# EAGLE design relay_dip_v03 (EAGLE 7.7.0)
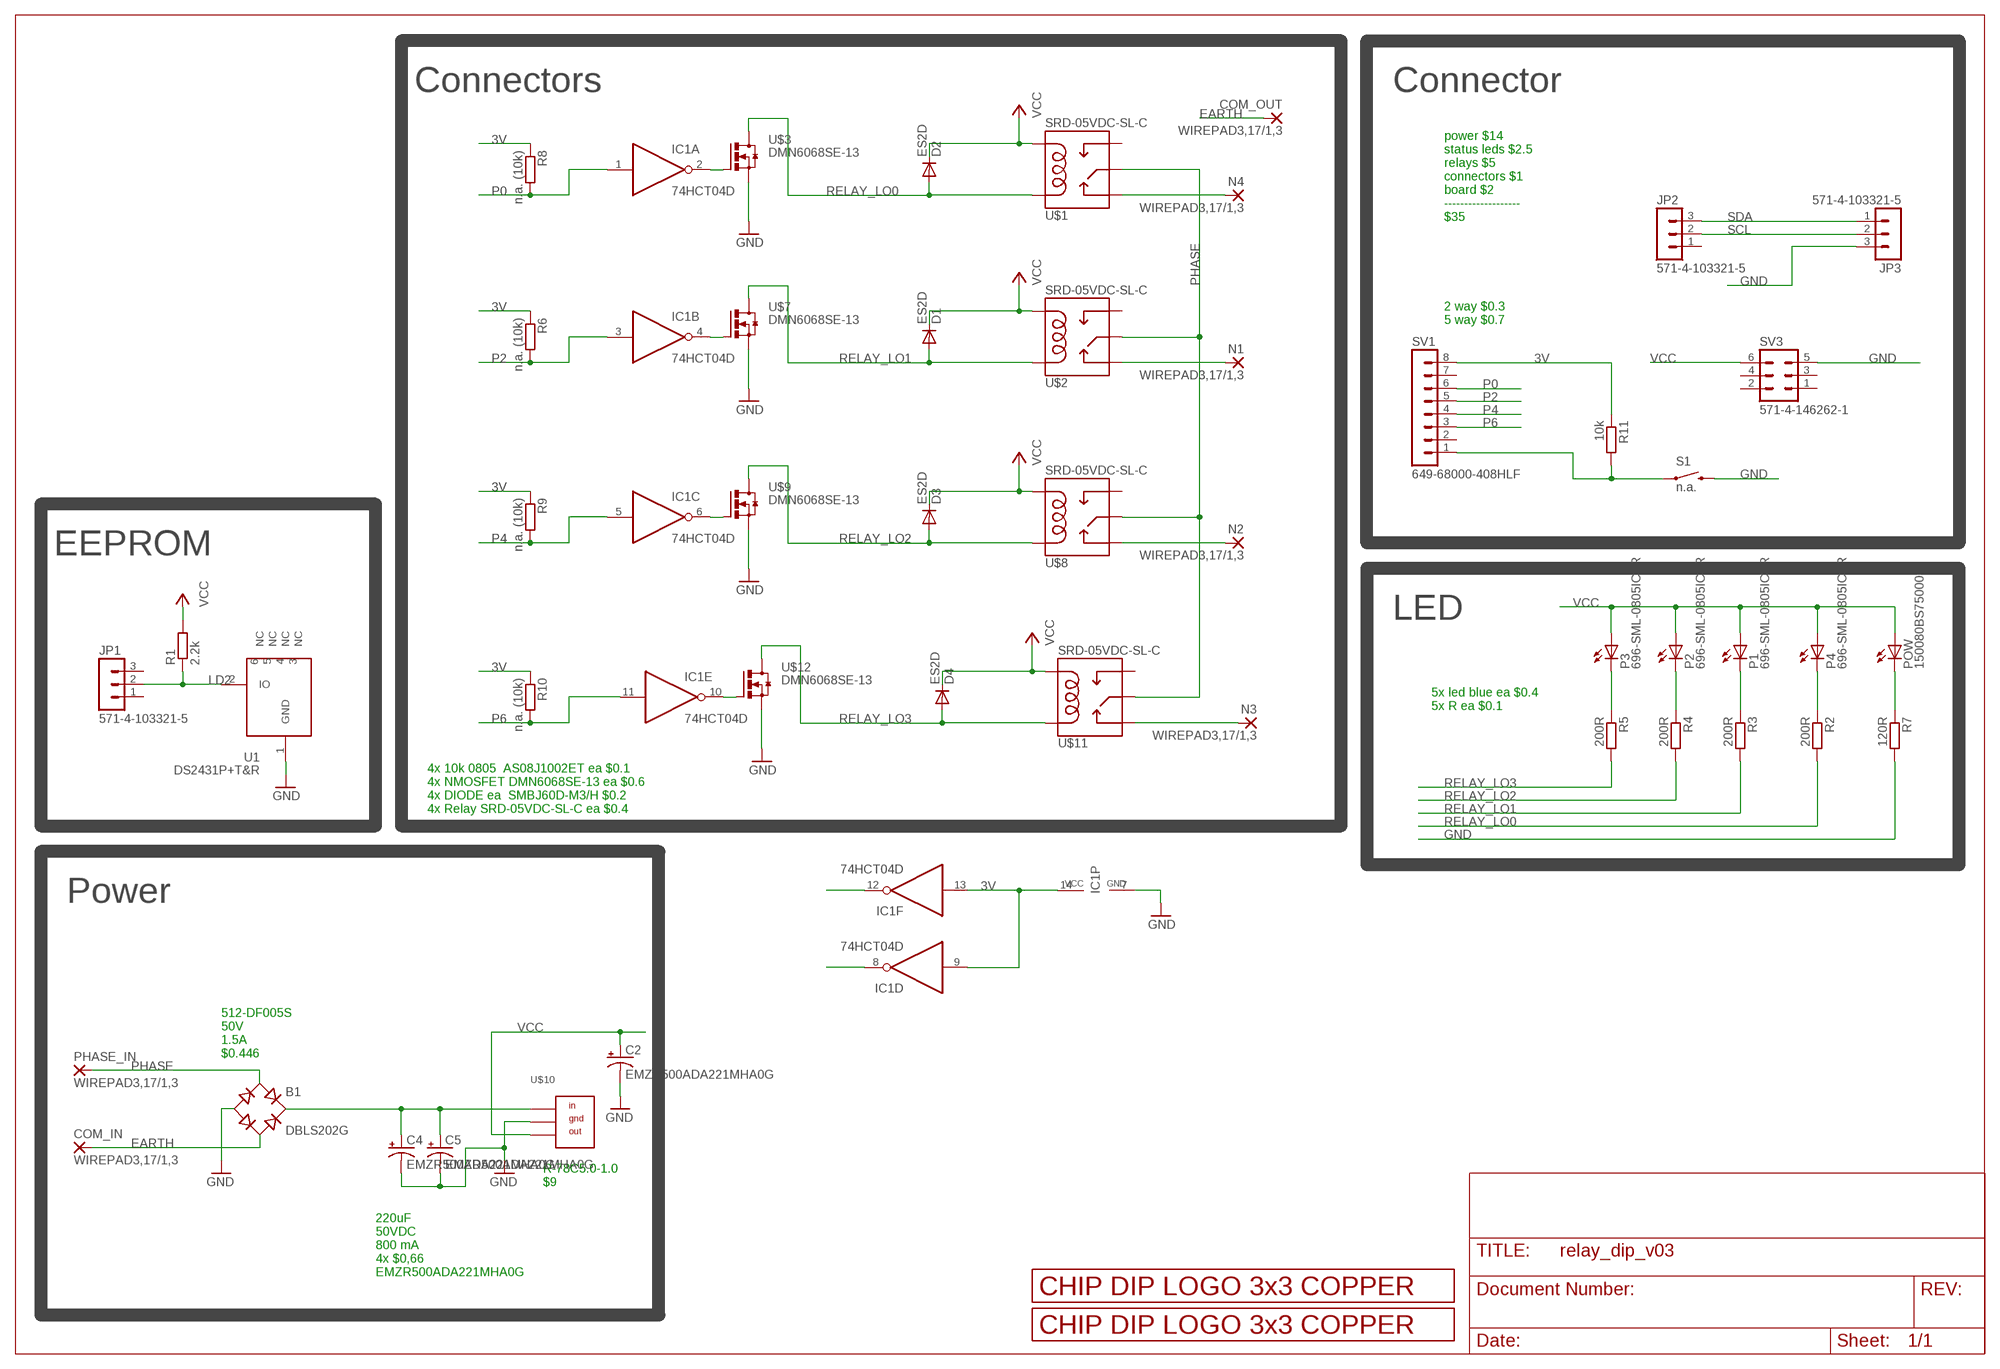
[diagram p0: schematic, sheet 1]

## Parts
B1  DBLS202G  [DBS]
C2  EMZR500ADA221MHA0G  CPOL-US150CLZ-0810  [150CLZ-0810]
C4  EMZR500ADA221MHA0G  CPOL-US150CLZ-0810  [150CLZ-0810]
C5  EMZR500ADA221MHA0G  CPOL-US150CLZ-0810  [150CLZ-0810]
COM_IN  WIREPAD3,17/1,3  [3,17/1,3]
COM_OUT  WIREPAD3,17/1,3  [3,17/1,3]
D1  ES2D  DIODE-SMB  [SMB]
D2  ES2D  DIODE-SMB  [SMB]
D3  ES2D  DIODE-SMB  [SMB]
D4  ES2D  DIODE-SMB  [SMB]
IC1  74HCT04D  [SO14]
JP1  571-4-103321-5  MA03-1  [MA03-1]
JP2  571-4-103321-5  MA03-1  [MA03-1]
JP3  571-4-103321-5  MA03-1  [MA03-1]
N1  WIREPAD3,17/1,3  [3,17/1,3]
N2  WIREPAD3,17/1,3  [3,17/1,3]
N3  WIREPAD3,17/1,3  [3,17/1,3]
N4  WIREPAD3,17/1,3  [3,17/1,3]
P1  696-SML-0805ICTR  LEDCHIP-LED0805  [CHIP-LED0805]
P2  696-SML-0805ICTR  LEDCHIP-LED0805  [CHIP-LED0805]
P3  696-SML-0805ICTR  LEDCHIP-LED0805  [CHIP-LED0805]
P4  696-SML-0805ICTR  LEDCHIP-LED0805  [CHIP-LED0805]
PHASE_IN  WIREPAD3,17/1,3  [3,17/1,3]
POW  150080BS75000  LEDCHIP-LED0805  [CHIP-LED0805]
R1  2.2k  R-EU_R0805  [R0805]
R2  200R  R-EU_R0805  [R0805]
R3  200R  R-EU_R0805  [R0805]
R4  200R  R-EU_R0805  [R0805]
R5  200R  R-EU_R0805  [R0805]
R6  n.a. (10k)  R-EU_R0805  [R0805]
R7  120R  R-EU_R0805  [R0805]
R8  n.a. (10k)  R-EU_R0805  [R0805]
R9  n.a. (10k)  R-EU_R0805  [R0805]
R10  n.a. (10k)  R-EU_R0805  [R0805]
R11  10k  R-EU_R0805  [R0805]
S1  n.a.  SWITCH-MOMENTARY-2SMD  [TACTILE-SWITCH-SMD]
SV1  649-68000-408HLF  MA08-1  [MA08-1]
SV3  571-4-146262-1  MA03-2  [MA03-2]
U1  DS2431P+T&R  DS2431P  [TSOC6]
U$1  SRD-05VDC-SL-C  RELAYPTH  [SRD-05VDC-SL-C]
U$2  SRD-05VDC-SL-C  RELAYPTH  [SRD-05VDC-SL-C]
U$3  DMN6068SE-13  NMOSFET_SMD_223  [SOT223]
U$4  LOGO_3X3_COPPER  [LOGO_3X3_COPPER]
U$6  LOGO_3X3_COPPER  [LOGO_3X3_COPPER]
U$7  DMN6068SE-13  NMOSFET_SMD_223  [SOT223]
U$8  SRD-05VDC-SL-C  RELAYPTH  [SRD-05VDC-SL-C]
U$9  DMN6068SE-13  NMOSFET_SMD_223  [SOT223]
U$10  R-7805-1.0  [SIP3]
U$11  SRD-05VDC-SL-C  RELAYPTH  [SRD-05VDC-SL-C]
U$12  DMN6068SE-13  NMOSFET_SMD_223  [SOT223]

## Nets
3V: IC1.9(D:I) IC1.13(F:I) IC1.14(P:VCC) R6.1 R8.1 R9.1 R10.1 R11.1 SV1.8
EARTH: B1.AC2 COM_IN.1(P) COM_OUT.1(P)
GND: B1.- C2.- C4.- C5.- IC1.7(P:GND) JP3.3 R7.2 S1.3 SV3.5 U1.1(GND) U$3.3(S) U$7.3(S) U$9.3(S) U$10.GND U$12.3(S)
LD2: JP1.2 R1.1 U1.2(IO)
N$1: R11.2 S1.1 SV1.1
N$2: IC1.2(A:O) U$3.1(G)
N$3: P4.C R2.1
N$4: P1.C R3.1
N$5: B1.+ C4.+ C5.+ U$10.IN
N$6: IC1.12(F:O)
N$7: IC1.4(B:O) U$7.1(G)
N$8: P2.C R4.1
N$9: IC1.6(C:O) U$9.1(G)
N$10: P3.C R5.1
N$11: IC1.10(E:O) U$12.1(G)
N$12: IC1.8(D:O)
N$29: POW.C R7.1
NCL: N4.1(P) U$1.SWCLOSED(SWCLOSE)
NCL1: N1.1(P) U$2.SWCLOSED(SWCLOSE)
NCL2: N2.1(P) U$8.SWCLOSED(SWCLOSE)
NCL3: N3.1(P) U$11.SWCLOSED(SWCLOSE)
P0: IC1.1(A:I) R8.2 SV1.6
P2: IC1.3(B:I) R6.2 SV1.5
P4: IC1.5(C:I) R9.2 SV1.4
P6: IC1.11(E:I) R10.2 SV1.3
PHASE: B1.AC1 PHASE_IN.1(P) U$1.SWCOMMON U$2.SWCOMMON U$8.SWCOMMON U$11.SWCOMMON
RELAY_LO0: D2.A R2.2 U$1.COIL1 U$3.2(D) U$3.4(D)
RELAY_LO1: D1.A R3.2 U$2.COIL1 U$7.2(D) U$7.4(D)
RELAY_LO2: D3.A R4.2 U$8.COIL1 U$9.2(D) U$9.4(D)
RELAY_LO3: D4.A R5.2 U$11.COIL1 U$12.2(D) U$12.4(D)
SCL: JP2.2 JP3.2
SDA: JP2.3 JP3.1
VCC: C2.+ D1.C D2.C D3.C D4.C P1.A P2.A P3.A P4.A POW.A R1.2 SV3.6 U$1.COIL0 U$2.COIL0 U$8.COIL0 U$10.OUT U$11.COIL0
Unconnected: JP1.1 JP1.3 JP2.1 SV1.2 SV1.7 SV3.1 SV3.2 SV3.3 SV3.4 U1.3(NC) U1.4(NC) U1.5(NC) U1.6(NC) U$1.SWOPEN U$2.SWOPEN U$8.SWOPEN U$11.SWOPEN

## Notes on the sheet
- Connectors | Connector
- power $14
  status leds $2.5
  relays $5
  connectors $1
  board $2
  -------------------
  $35
- 2 way $0.3
  5 way $0.7
- EEPROM
- LED
- 5x led blue ea $0.4
  5x R ea $0.1
- 4x 10k 0805  AS08J1002ET ea $0.1
  4x NMOSFET DMN6068SE-13 ea $0.6
  4x DIODE ea  SMBJ60D-M3/H $0.2
  4x Relay SRD-05VDC-SL-C ea $0.4
- Power
- 512-DF005S
  50V
  1.5A
  $0.446
- R-78C5.0-1.0
  $9
- 220uF
  50VDC
  800 mA
  4x $0,66
  EMZR500ADA221MHA0G

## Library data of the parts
B1 = rectifier:DB?*G: Single Phase 1.0 AMP Glass Passivated Bridge Rectifier Taiwan Semiconductor Co.,Ltd. - TSC Source: http://www.taiwansemi.com/TSCbig5/ezcatfiles/cust/img/img/db101g.pdf http://www.ts.com.tw/db/pictures/modules/PDT/PDT060207001/DBLS201G.pdf
C2 C4 C5 = rcl:CPOL-US: POLARIZED CAPACITOR, American symbol
COM_IN COM_OUT N1-N4 PHASE_IN = wirepad:WIREPAD: Wire PAD connect wire on PCB
D1-D4 = diode:DIODE-: DIODE
IC1 = 74xx-eu:74*04: Hex INVERTER
JP1-JP3 = con-lstb:MA03-1: PIN HEADER; OC_FARNELL: unknown; OC_NEWARK: unknown
P1-P4 POW = led:LED: LED
R1-R11 = rcl:R-EU_: RESISTOR, European symbol
S1 = SparkFun-Electromechanical:SWITCH-MOMENTARY-2: Various NO switches- pushbuttons, reed, etc; PROD_ID: SWCH-08247
SV1 = con-lstb:MA08-1: PIN HEADER; OC_FARNELL: unknown; OC_NEWARK: unknown
SV3 = con-lstb:MA03-2: PIN HEADER; OC_FARNELL: unknown; OC_NEWARK: unknown
U1 = JKW_CHIP:DS2431: 1024-Bit EEPROM This chip provides a 4x256 Bit EEPROM, which can be programmed@5V. Write protection and OTP emulation are available, too. Author: Jan Kandziora <jjj@gmx.de>; DESCRIPTION: IC, 1024-Bit, 1-Wire EEPROM, TSOC6; FOOTPRINT: TSOC6; LINK: http://www.digikey.com/product-detail/en/DS2431P%2BT%26R/DS2431P%2BT%26RCT-ND/3647900; MFG: DIGIKEY; MFG_PN: DS2431P+T&RCT-ND; PART_TYPE: IC; PRICE: 0.98; VENDOR: MAXIM; VENDOR_PART_NUMBER: DS2431P+T&R
U$1 U$2 U$8 U$11 = SRD-05VDC-SL-C:RELAY: SPDT relay (COM-00101)
U$3 U$7 U$9 U$12 = transistor-power:NMOSFET_SMD_223
U$4 U$6 = logo:LOGO_3X3_COPPER
U$10 = Kolja:R-7805-1.0

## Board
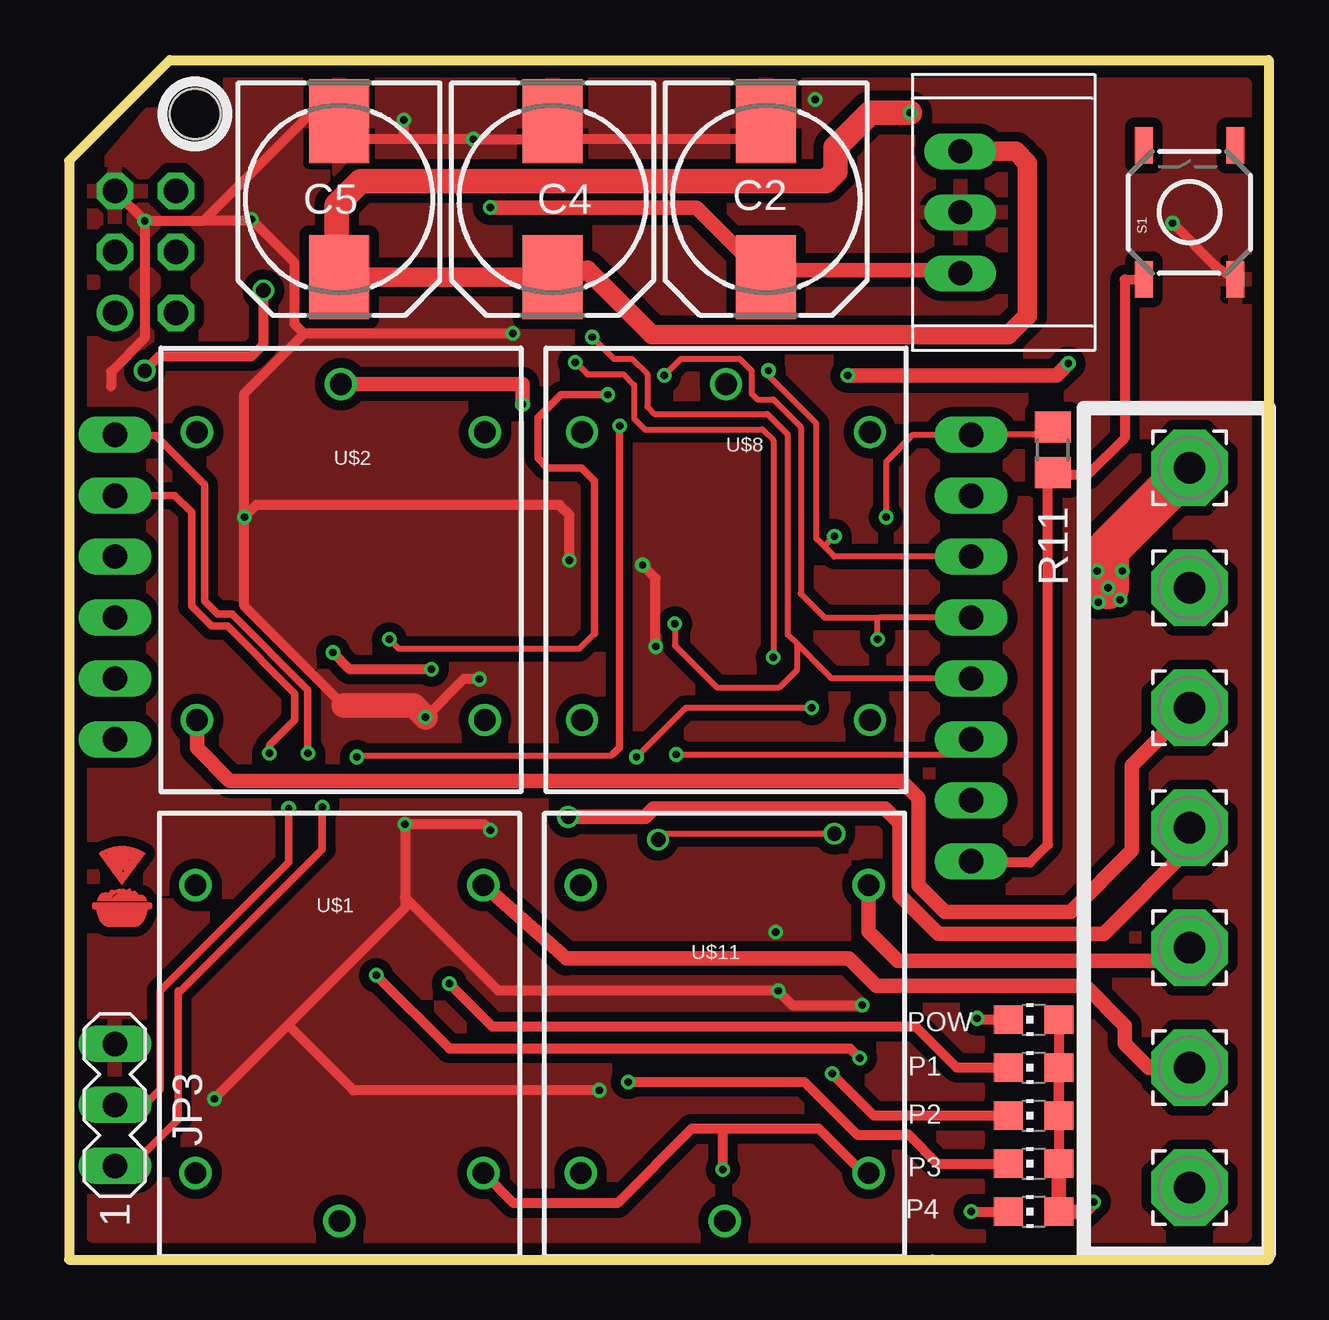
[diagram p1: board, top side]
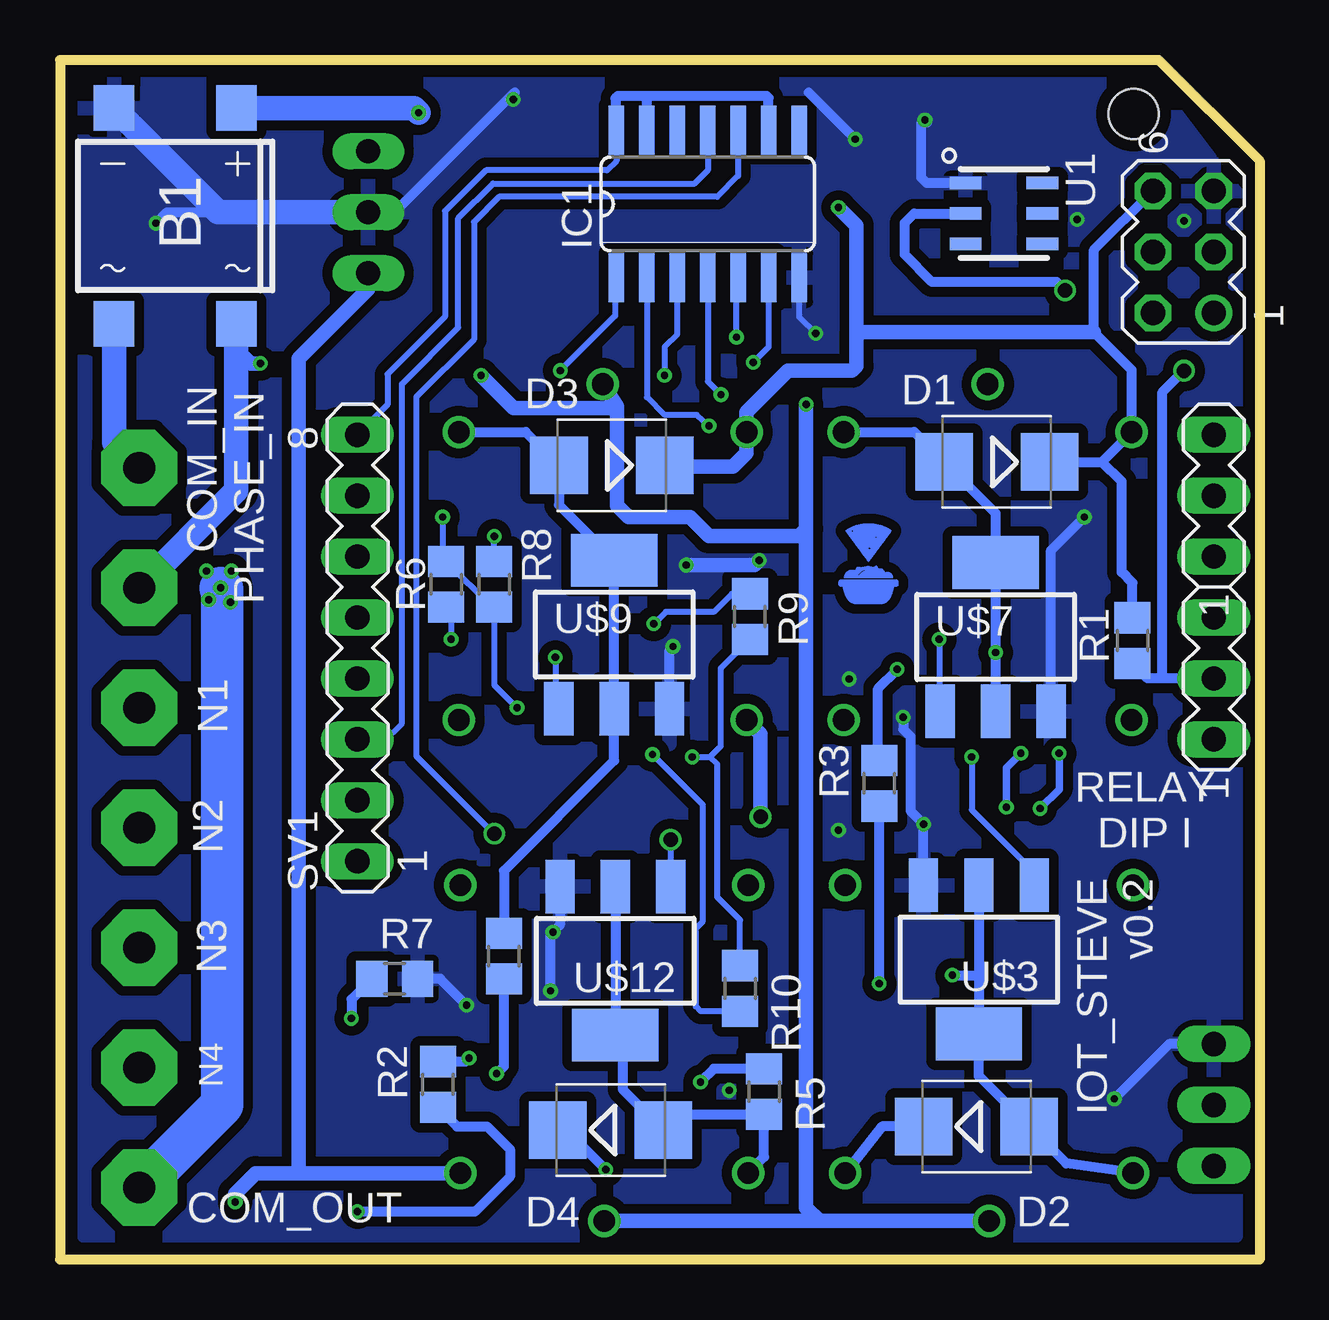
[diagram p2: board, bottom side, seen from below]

Size 50 x 50 mm. Coordinates in mm from the lower left corner, seen from the top.
Outline: 4.2,50 50,50 50,0 0,0 0,45.8 4.2,50
Copper layers (1*16): Top 0.035mm / dielectric 1.6mm / Bottom 0.035mm
Design rules "Elecrow_2-layer_PCB_eagle_rule": minimum track width 6mil, minimum drill 12mil, track to track 6mil, track to pad 6mil, pad to pad 6mil, via to via 8mil, smd to smd 0mil, copper to edge 20mil, drill to drill 10mil, minimum pad ring 6mil, minimum via ring 6mil, stop-mask expansion 0mil, vias tented up to drill 100mil, thermal gap 10mil
Holes 2.1 mm at 5.25,47.75

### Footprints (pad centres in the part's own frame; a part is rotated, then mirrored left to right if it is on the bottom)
DBS = smd 1.7 x 1.9: + -2.55,-4.5; - 2.55,-4.5; AC1 -2.55,4.5; AC2 2.55,4.5
150CLZ-0810 = smd 3.5 x 2.5: + 3.25,0; - -3.25,0
3,17/1,3 = drill 1.321 pad 3.175 octagon: 1 0,0
SMB = smd 2.4 x 2.4: A 2.2,0; C -2.2,0
SO14 = smd 0.66 x 2.032: 1 -3.81,-3.073; 2 -2.54,-3.073; 3 -1.27,-3.073; 4 0,-3.073; 5 1.27,-3.073; 6 2.54,-3.073; 7 3.81,-3.073; 8 3.81,3.073; 9 2.54,3.073; 10 1.27,3.073; 11 0,3.073; 12 -1.27,3.073; 13 -2.54,3.073; 14 -3.81,3.073
MA03-1 = drill 1.016 long: 1 -2.54,0; 2 0,0; 3 2.54,0
CHIP-LED0805 = smd 1.2 x 1.2: A 0,-1.05; C 0,1.05
R0805 = smd 1.3 x 1.5: 1 -0.95,0; 2 0.95,0
TACTILE-SWITCH-SMD = smd 1.524 x 0.762: 1 -2.794,1.905; 2 2.794,1.905; 3 -2.794,-1.905; 4 2.794,-1.905
MA08-1 = drill 1.016 long: 1 -8.89,0; 2 -6.35,0; 3 -3.81,0; 4 -1.27,0; 5 1.27,0; 6 3.81,0; 7 6.35,0; 8 8.89,0
MA03-2 = drill 1.016: 1 -2.54,-1.27 | drill 1.016 octagon: 2 -2.54,1.27; 3 0,-1.27; 4 0,1.27; 5 2.54,-1.27; 6 2.54,1.27
TSOC6 = smd 0.53 x 1.33: 1 -1.27,-1.6; 2 0,-1.6; 3 1.27,-1.6; 4 1.27,1.6; 5 0,1.6; 6 -1.27,1.6
SRD-05VDC-SL-C = drill 0.9: COIL0 -5.39,-6.12; COIL1 -5.39,5.88; SWCLOSED 6.61,-6.12; SWCOMMON -7.39,-0.12; SWOPEN 6.61,5.88
SOT223 = smd 1.219 x 2.235: 1 -2.311,-3.099; 2 0,-3.099; 3 2.311,-3.099 | smd 3.6 x 2.2: 4 0,3.099
SIP3 = drill 1 long: GND 5.75,2; IN 3.21,2; OUT 8.29,2

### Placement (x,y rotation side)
B1  45.2,43.5 180 bottom
C2  29.05,44.2 270 top
C4  20.15,44.2 270 top
C5  11.25,44.2 270 top
COM_IN  46.7,33 90 top
COM_OUT  46.7,3 90 top
D1  10.95,33.25 180 bottom
D2  11.8,5.55 0 bottom
D3  27,33.1 180 bottom
D4  27.05,5.4 0 bottom
IC1  23,44 0 bottom
JP1  1.91,24.22 90 bottom
JP2  1.91,31.84 90 bottom
JP3  1.91,6.44 90 top
N1  46.7,23 0 top
N2  46.7,18 0 top
N3  46.7,13 0 top
N4  46.7,8 90 top
P1  40.2,8 90 top
P2  40.2,6 90 top
P3  40.2,4 90 top
P4  40.2,2 90 top
PHASE_IN  46.7,28 90 top
POW  40.2,10 90 top
R1  5.3,25.8 90 bottom
R2  34.25,7.3 90 bottom
R3  15.85,19.85 90 bottom
R4  31.5,12.65 90 bottom
R5  20.65,7 270 bottom
R6  33.9,28.15 270 bottom
R7  36.05,11.7 0 bottom
R8  31.9,28.15 90 bottom
R9  21.25,26.8 90 bottom
R10  21.65,11.3 270 bottom
R11  41,33.75 270 top
S1  46.7,43.65 90 top
SV1  37.6,25.49 90 bottom
SV3  3.17,42 90 bottom
U1  10.65,43.6 270 bottom
U$1  11.15,9 90 top
U$2  11.45,29.1 270 top
U$3  11.7,12.5 180 bottom
U$4  2.2,15.55 0 top
U$6  16.3,29 0 bottom
U$7  11,25.95 0 bottom
U$8  27.5,29.1 270 top
U$9  26.9,26.05 0 bottom
U$10  35.15,49.4 270 top
U$11  27.2,9 90 top
U$12  26.85,12.45 180 bottom

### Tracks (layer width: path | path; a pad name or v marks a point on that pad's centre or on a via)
3V  (via drill 0.3)
  Top 0.254: v34.05,30.95 34.05,33.25 35.18,34.38 SV1.8 40.68,34.38 | v30.95,23 25.7,23 v23.65,20.95
  Top 0.406: 40.68,34.38 R11.1
  Bottom 0.254: IC1.14 26.81,45.79 27.2,45.4 32.25,45.4 33.95,43.7 33.95,39.3 36.35,36.9 36.35,35.63 SV1.8 | v34.05,30.95 34.05,29.25 R6.1 32,27.2 R8.1 31.9,23.95 v30.95,23 | v23.65,20.95 22.9,20.95 | 22.9,20.95 22.45,21.4 22.45,24.65 R9.1 | R10.1 21.65,14.15 22.6,15.1 22.6,20.65 22.9,20.95
  Bottom 0.406: IC1.9 20.46,48.41 20.55,48.5 25.6,48.5 | 25.6,48.5 26.75,48.5 26.85,48.4 26.85,47.11 IC1.14 | IC1.13 25.54,48.44 25.6,48.5
EARTH  (via drill 0.3)
  Top 1.778: v43.3,28 43.3,29.6 COM_IN.1
  Bottom 0.406: v42.9,27.4 42.9,27.6 v43.3,28 | v43.3,28 43.3,28.1 | 43.3,28.1 v43.9,28.7 | v43.8,27.5 v43.3,28 | 43.3,28.1 43.3,28.25 v42.85,28.7
  Bottom 0.813: 45.7,3 COM_OUT.1
  Bottom 1.016: B1.AC2 47.75,34.05 COM_IN.1
  Bottom 1.778: COM_OUT.1 43.25,6.45 43.25,27.95 v43.3,28
GND  (via drill 0.3)
  Top 0.406: v3.15,43.3 3.19,43.25 3.29,43.35 3.35,43.3 5.6,43.3 | v3.15,43.3 3.15,38.4 1.75,37 1.75,36.4 | 11.45,23.1 7.3,27.25 v7.3,30.95 | v33.05,10.6 30.15,10.6 v29.55,11.2 17.9,11.2 14,15.1 | 5.6,43.3 10.05,47.75 C5.- 12.3,46.7 14,46.7 | 19.1,46.7 v16.85,46.7 14,46.7 | 19.1,46.7 C4.- | v13.95,47.5 13.95,46.75 14,46.7 | 5.6,43.3 7.55,43.3 v7.6,43.35 9.4,41.55 9.4,39 9.8,38.6 | v18.5,38.6 9.8,38.6 | v7.3,30.95 7.3,36.1 9.8,38.6 | v17.55,17.9 17.3,18.15 v14,18.15 14,15.1 | 14,15.1 14,14.65 9.12,9.78 | 9.12,9.78 v6.05,6.7 | v22.1,7.05 11.85,7.05 9.12,9.78 | v24.45,25.55 24.45,28.4 v23.9,28.95 | v17.1,24.2 16.45,24.2 v14.85,22.6 | v20.85,29.15 20.85,31.05 20.45,31.45 7.8,31.45 v7.3,30.95 | S1.3 47.8,41.4 v46,43.2 | C2.- 28,46.7 19.1,46.7 | SV3.5 v3.15,43.3
  Top 1.016: v14.85,22.6 14.35,23.1 11.45,23.1
  Bottom 0.254: IC1.7 19.19,39.29 v18.5,38.6
  Bottom 0.406: U$10.GND 36.05,43.65 31.05,48.65 | 18.8,48.65 v16.85,46.7 | 13.85,47.4 v13.95,47.5 14.1,47.35 14.1,45.1 13.87,44.87 U1.1 | v14.85,22.6 14.85,22.1 14.55,21.8 14.55,18.7 14.01,18.16 | 14.01,18.16 v14,18.15 | JP3.3 3.77,8.98 v6.05,6.7 | U$3.3 14.01,18.16 | v29.55,11.2 29.55,13.55 v29.45,13.65 29.16,13.94 U$12.3 | U$9.3 24.59,25.41 v24.45,25.55 | 21.05,28.95 v20.85,29.15 | U$7.3 8.69,29.56 v7.3,30.95 | v46,43.2 45.55,43.65 43.25,43.65 | v33.05,10.6 34.15,11.7 R7.2
  Bottom 0.61: 20.9,29.1 21.05,28.95 v23.9,28.95
  Bottom 1.016: B1.- 43.4,43.65 43.25,43.65 U$10.GND
  other vias: 31.1,48.35
  pour Top (isolate 0.406): 1,1 1,45 4.4,49 49,49 49,1
  pour Bottom (isolate 0.406): 1,1 49,1 49,49 4.4,49 1,44.5
LD2  (via drill 0.6)
  Top 0.406: v3.15,37.05 3.75,37.65 7.6,37.65 8.1,38.15 v8.1,40.4
  Bottom 0.406: JP1.2 4.2,24.22 | 4.2,24.22 4.67,24.22 R1.1 | 4.2,24.22 4.05,24.37 4.05,36.15 v3.15,37.05 | v8.1,40.4 8.45,40.75 13.65,40.75 14.8,41.9 14.8,43.2 14.4,43.6 U1.2
N$1
  Top 0.254: 37.65,16.55 SV1.1
  Top 0.406: 37.65,16.55 40.05,16.55 40.8,17.3 40.8,32.6 R11.2 41.1,32.7 42.45,32.7 44,34.25 44,40.85 S1.1
N$2  (via drill 0.3)
  Top 0.254: 22.7,21.1 22.6,21 12.05,21 v12,20.95
  Top 0.305: 22.7,21.1 22.95,21.35 v22.95,34.75
  Bottom 0.254: IC1.2 25.54,35.94 24.8,35.2 23.45,35.2 v22.95,34.75 | v12,20.95 12,18.75 9.39,16.14 U$3.1
N$3  (via drill 0.3)
  Top 0.406: v37.6,2 P4.C
  Bottom 0.406: R2.1 33.45,5.55 32.2,5.55 31.25,4.6 31.25,3.45 32.7,2 v37.6,2
N$4  (via drill 0.3)
  Top 0.406: P1.C 37,8 35.3,9.7 17.65,9.7 v15.85,11.5
  Bottom 0.406: v15.85,11.5 R3.1
N$5  (via drill 0.3)
  Top 0.813: C5.+ C4.+ 21.6,41.25 24.3,38.55 39.15,38.55 39.95,39.35 39.95,45.7 39.46,46.19 U$10.IN
  Top 1.016: v35.05,47.8 33.4,47.8 31.95,46.35 31.95,45.35 31.55,44.95 12.15,44.95 11.15,43.95 11.15,41.35 C5.+
  Bottom 1.016: B1.+ 35.25,48 v35.05,47.8
N$7  (via drill 0.3)
  Top 0.254: 21.9,26.1 21.25,25.45 13.75,25.45 v13.35,25.85
  Top 0.305: 21.9,26.1 21.9,32.45 21.35,33 19.95,33 19.55,33.4 19.55,35.1 20.5,36.05 v22.45,36.05
  Bottom 0.254: IC1.4 23,36.6 v22.45,36.05 | v13.35,25.85 13.35,22.89 U$7.1
N$8  (via drill 0.3)
  Top 0.406: P2.C 33.55,6 v31.8,7.75
  Bottom 0.406: v31.8,7.75 31.5,8.05 R4.1
N$9  (via drill 0.3)
  Top 0.254: v21.1,37.4 21.6,36.9 23.1,36.9 23.55,36.45 23.55,35.05 24,34.6 28.9,34.6 29.35,34.15 v29.35,25.1
  Bottom 0.254: IC1.6 20.46,38.04 v21.1,37.4 | v29.35,25.1 29.35,23.09 U$9.1
N$10  (via drill 0.3)
  Top 0.406: v23.3,7.4 30.65,7.4 32.85,5.2 35,5.2 36.2,4 P3.C
  Bottom 0.406: R5.1 22.75,7.95 v23.3,7.4
N$11  (via drill 0.6)
  Top 0.254: v31.9,17.75 24.8,17.75 v24.55,17.5
  Bottom 0.254: v24.55,17.5 U$12.1 | IC1.10 21.73,45.17 22.6,44.3 31.7,44.3 32.75,43.25 32.75,38.35 35.15,35.95 35.15,21 v31.9,17.75
N$29  (via drill 0.3)
  Top 0.406: POW.C 37.9,10 v37.85,10.05
  Bottom 0.406: R7.1 37.85,10.85 v37.85,10.05
NCL
  Top 0.61: N4.1 45,8 44,9 44,9.75 42.35,11.4 33.65,11.4 32.5,12.55 20.73,12.55 U$1.SWCLOSED
NCL1
  Top 0.61: U$2.SWCLOSED 5.33,21.32 6.7,19.95 34.7,19.95 35.4,19.25 35.4,15.6 36.5,14.5 41.75,14.5 44.3,17.05 44.3,20.6 N1.1
NCL2  (via drill 0.6)
  Top 0.61: v20.8,18.45 24,18.45 24.35,18.8 34,18.8 34.6,18.2 34.6,15.2 36.23,13.57 43.12,13.57 46.7,17.15 N2.1
  Bottom 0.61: v20.8,18.45 20.8,21.91 U$8.SWCLOSED
NCL3
  Top 0.61: N3.1 46.15,12.45 34.55,12.45 33.32,13.68 U$11.SWCLOSED
P0  (via drill 0.3)
  Top 0.254: 31.43,29.77 31.15,30.05 31.15,34.85 29.15,36.85 v29.15,37.05 | v31.9,30.15 31.52,29.77 31.43,29.77 | SV1.6 31.9,29.3 31.43,29.77
  Bottom 0.254: R8.2 v31.9,30.15 | v29.15,37.05 26.86,39.34 26.86,40.88 IC1.1
P2  (via drill 0.3)
  Top 0.254: v33.7,25.85 33.7,26.7 | 33.7,26.7 33.7,26.76 31.49,26.76 30.5,27.75 30.5,34.7 29.35,35.85 28.7,35.85 28.45,36.1 28.45,37.05 27.95,37.55 25.5,37.55 v24.8,36.85 | SV1.5 33.76,26.76 33.7,26.7
  Bottom 0.254: IC1.3 24.27,38.58 24.8,38.05 v24.8,36.85 | R6.2 33.7,27 v33.7,25.85
P4  (via drill 0.3)
  Top 0.254: 30.35,25.65 29.95,26.05 29.95,34.4 29.1,35.25 24.4,35.25 24.1,35.55 24.1,36.9 23.45,37.55 22.7,37.55 v21.8,38.45 | 30.35,25.65 31.55,24.45 31.78,24.22 SV1.4 | v25.25,26.5 25.25,25.6 27,23.85 29.6,23.85 30.35,24.6 30.35,25.65
  Bottom 0.254: v21.8,38.45 21.8,40.86 IC1.5 | R9.2 22,27.75 22.75,27 24.75,27 v25.25,26.5
P6  (via drill 0.3)
  Top 0.254: v25.3,21.05 36.97,21.05 SV1.3
  Bottom 0.254: IC1.11 23,45.4 23.55,44.85 31.95,44.85 33.4,43.4 33.4,38.85 35.75,36.5 35.75,22.35 36.55,21.55 37.47,21.55 SV1.3 | R10.2 23.3,10.35 23.5,10.55 23.5,13.8 23.2,14.1 23.2,18.95 v25.3,21.05
PHASE  (via drill 0.3)
  Top 0.61: U$2.SWCOMMON 18.9,36.49 v18.9,35.65 | v32.45,36.85 41.15,36.85 v41.65,37.35
  Bottom 0.61: 18.9,30.45 18.9,2.16 18.35,1.61 | 18.9,30.45 v18.9,35.65 | U$8.SWCOMMON 26.78,35.55 | 26.78,35.55 26.78,31.43 26.3,30.95 23.75,30.95 22.95,30.15 19.2,30.15 18.9,30.45 | v32.45,36.85 31.1,35.5 26.83,35.5 26.78,35.55 | v41.65,37.35 42.05,37.35 42.65,37.95 | U$1.SWCOMMON 18.35,1.61 | U$11.SWCOMMON 18.35,1.61
  Bottom 1.016: B1.AC1 42.65,37.95 42.65,32.05 PHASE_IN.1
RELAY_LO0  (via drill 0.3)
  Top 0.406: v12.8,11.85 15.85,8.8 32.55,8.8 v32.95,8.4
  Bottom 0.406: U$3.2 11.7,11.85 | 11.7,11.85 U$3.4 11.7,7.65 D2.A 8.06,4.01 U$1.COIL1 | v12.8,11.85 11.7,11.85 | v32.95,8.4 33.1,8.25 R2.2
RELAY_LO1  (via drill 0.3)
  Top 0.406: v15.1,24.6 11.7,24.6 v11,25.3
  Bottom 0.406: U$2.COIL1 14.39,34.49 D1.A 11,31.1 U$7.4 v11,25.3 U$7.2 10.95,22.8 | v15.1,24.6 15.9,23.8 15.9,20.85 R3.2
RELAY_LO2
  Bottom 0.406: U$8.COIL1 30.59,34.49 D3.A 29.2,31.45 U$9.4 U$9.2 26.9,20.8 31.5,16.2 R4.2
RELAY_LO3
  Bottom 0.406: U$12.2 U$12.4 | U$12.4 26.85,9.2 26.55,8.9 26.55,7.1 D4.A 24.2,6.05 R5.2 | 27.2,9 U$12.4 | R5.2 20.72,5.98 | U$11.COIL1 20.65,4.28 R5.2
SCL  (via drill 0.3)
  Top 0.305: JP3.2 3.15,6.45 3.8,7.1 3.8,11.2 9.15,16.55 v9.15,18.8 | JP2.2 4.41,31.84 5.1,31.15 5.1,27.25 5.95,26.4 6.6,26.4 9.4,23.6 9.4,22.5 8.35,21.45 v8.35,21.1
  Bottom 0.305: v8.35,21.1 8.35,19.6 v9.15,18.8
SDA  (via drill 0.3)
  Top 0.305: JP3.1 2.6,3.9 4.55,5.85 4.55,11.2 4.65,11.2 10.55,17.1 v10.55,18.85 | v9.95,21.1 9.95,23.75 6.8,26.9 6.2,26.9 5.65,27.45 5.65,32.3 3.6,34.35 1.94,34.35 JP2.3
  Bottom 0.305: v10.55,18.85 10.55,20.5 v9.95,21.1
VCC  (via drill 0.3)
  Top 0.406: POW.A P1.A | P2.A P1.A | P1.A P3.A | 27.1,5.45 31.25,5.45 33.09,3.61 U$11.COIL0 | 27.1,5.45 25.95,5.45 22.85,2.35 18.53,2.35 U$1.COIL0 | v27.25,3.75 27.25,5.3 27.1,5.45
  Top 0.61: U$10.OUT 37.01,41.25 29.35,41.25 C2.+ 26.15,43.85 v17.55,43.85 | P3.A P4.A 42.3,2 v42.7,2.4
  Bottom 0.406: 24.75,33.05 D3.C | D1.C 6.57,33.25 | 6.57,33.25 U$2.COIL0 5.33,37.08 6.9,38.65 6.9,42.09 SV3.6 | D2.C 15.73,5.55 U$1.COIL0 | D4.C 28.9,5.4 v27.25,3.75 | R1.2 5.3,28.2 5.75,28.65 5.75,32.43 6.57,33.25
  Bottom 0.61: 6.9,38.65 16.75,38.65 16.8,38.7 | 40.15,3.6 41.85,3.6 42.7,2.75 v42.7,2.4 | 40.15,3.6 33.13,3.6 U$11.COIL0 | v17.55,43.85 16.8,43.1 16.8,38.7 | 16.8,38.7 16.8,37.25 17,37.05 19.65,37.05 21.38,35.32 U$8.COIL0 21.38,33.62 21.95,33.05 24.75,33.05 | U$10.OUT 37.15,40.45 40.05,37.55 40.05,3.7 40.15,3.6

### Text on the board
bPlace: RELAY / DIP I | IOT_STEVE / v0.2

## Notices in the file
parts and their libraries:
SparkFun-Electromechanical: Licensing: Creative Commons ShareAlike 4.0 International - https://creativecommons.org/licenses/by-sa/4.0
